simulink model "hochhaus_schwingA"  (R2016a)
settings: Solver=ode45  StartTime=0.0  StopTime=1000  MaxStep=1e-3  RelTol=1e-3
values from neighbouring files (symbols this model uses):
  m = 1.0    (= 1)    [init_pendelStange.m]
undefined symbols (not defined in the file or in its folder): v0, x0
libraries: simulink x1, simulink_extras x1

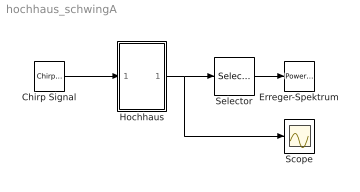
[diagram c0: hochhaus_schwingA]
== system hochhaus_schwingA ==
  Chirp Signal : simulink/Sources/Chirp Signal  f1=5/(2*pi)  T=1000  f2=50/(2*pi)
  Erreger-Spektrum : simulink_extras/Additional Sinks/Power Spectral Density  npts=2048  fftpts=2048  HowOften=64  sampleT=0.05
  Hochhaus : Subsystem
  Scope : Scope
  Selector : Selector  InputPortWidth=3  IndexOptions=Index vector (dialog)  Indices=[3]  OutputSizes=1
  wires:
  Hochhaus/1(x) -> Selector/1, Scope/1
  Chirp Signal/1 -> Hochhaus/1(F)
  Selector/1 -> Erreger-Spektrum/1

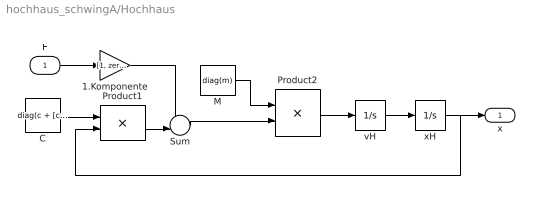
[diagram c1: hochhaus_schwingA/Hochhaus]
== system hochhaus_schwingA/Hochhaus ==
  F : Inport
  1.Komponente : Gain  Gain=[1, zeros(1,length(m)-1)]
  C : Constant  Value=diag(c + [c(2:end),0]) - diag(c(2:end),1) - diag(c(2:end),-1)  VectorParams1D=off
  M : Constant  Value=diag(m)  VectorParams1D=off
  Product1 : Product  Multiplication=Matrix(*)
  Product2 : Product  Inputs=/*  Multiplication=Matrix(*)
  Sum : Sum  Inputs=+-|
  vH : Integrator  InitialCondition=v0
  xH : Integrator  InitialCondition=x0
  x : Outport
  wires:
  1.Komponente/1 -> Sum/1
  F/1 -> 1.Komponente/1
  M/1 -> Product2/1
  Product2/1 -> vH/1
  Sum/1 -> Product2/2
  C/1 -> Product1/1
  Product1/1 -> Sum/2
  xH/1 -> x/1, Product1/2
  vH/1 -> xH/1
